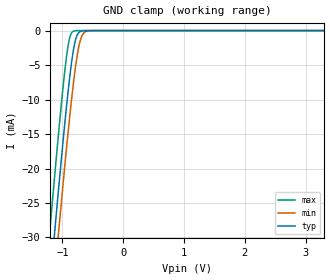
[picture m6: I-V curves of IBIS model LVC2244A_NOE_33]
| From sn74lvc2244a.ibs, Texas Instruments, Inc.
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[Model]   LVC2244A_NOE_33
Model_type  Input
Vinl=0.8
Vinh=2.0
| variable   typ   min   max
C_comp   5.21pF   4.78pF   5.55pF
[Temperature Range]   40   100   -40
| Ambient temperature   25   85   -40
[Voltage range]   3.3   3   3.6
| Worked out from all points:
|   GND clamp passes 1 mA (typ) near -0.77 V on its own axis
[GND Clamp]
| LVC2244A_NOE_33
|   Voltage   I(typ)   I(min)   I(max)
-5V       -443mA     -448.4mA   -436.3mA
-1.21V    -37.44mA   -43.78mA   -29.29mA
-1.135V   -29.95mA   -36.3mA    -21.79mA
-1.115V   -27.98mA   -34.33mA   -19.83mA
-1.055V   -22.16mA   -28.48mA   -14.08mA
-915mV    -9.525mA   -15.47mA   -2.668mA
-870mV    -6.037mA   -11.62mA   -738.2uA
-815mV    -2.628mA   -7.333mA   -73.84uA
-765mV    -815.6uA   -4.067mA   -7.221uA
-710mV    -147.1uA   -1.578mA   -543.8nA
-585mV    -1.929uA   -60.17uA   -1.522nA
3.3V      9.498pA    15.54pA    9.116pA
